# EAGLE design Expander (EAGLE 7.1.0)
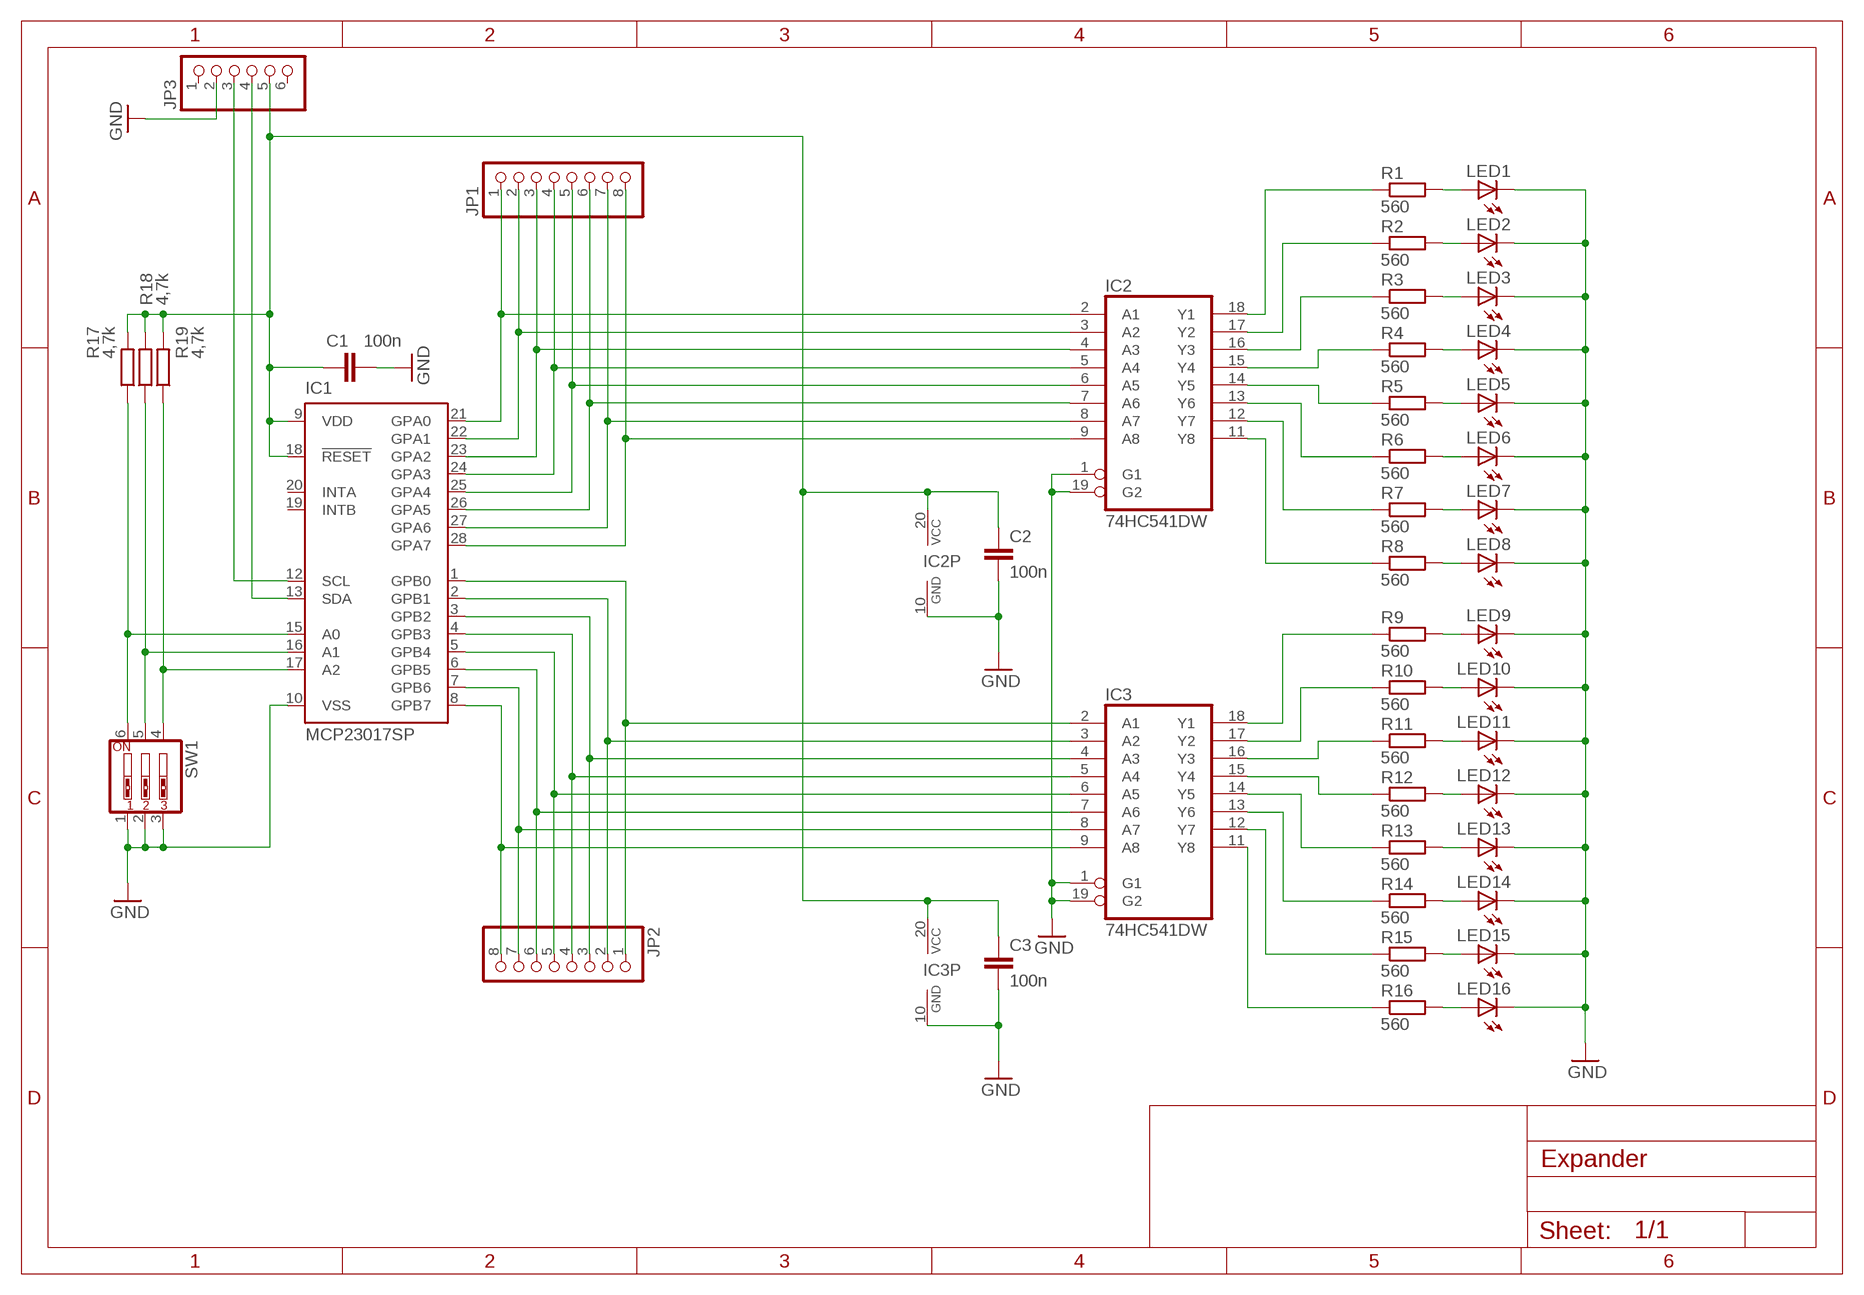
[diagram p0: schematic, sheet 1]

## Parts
C1  100n  C-EUC1206  [C1206]
C2  100n  C-EUC1206  [C1206]
C3  100n  C-EUC1206  [C1206]
IC1  MCP23017SP  [DIL28-3]
IC2  74HC541DW  [SO20W]
IC3  74HC541DW  [SO20W]
JP1  PINHD-1X8  [1X08]
JP2  PINHD-1X8  [1X08]
JP3  PINHD-1X6/90  [1X06/90]
LED1  LEDSMT1206  [1206]
LED2  LEDSMT1206  [1206]
LED3  LEDSMT1206  [1206]
LED4  LEDSMT1206  [1206]
LED5  LEDSMT1206  [1206]
LED6  LEDSMT1206  [1206]
LED7  LEDSMT1206  [1206]
LED8  LEDSMT1206  [1206]
LED9  LEDSMT1206  [1206]
LED10  LEDSMT1206  [1206]
LED11  LEDSMT1206  [1206]
LED12  LEDSMT1206  [1206]
LED13  LEDSMT1206  [1206]
LED14  LEDSMT1206  [1206]
LED15  LEDSMT1206  [1206]
LED16  LEDSMT1206  [1206]
R1  560  R-EU_R1206  [R1206]
R2  560  R-EU_R1206  [R1206]
R3  560  R-EU_R1206  [R1206]
R4  560  R-EU_R1206  [R1206]
R5  560  R-EU_R1206  [R1206]
R6  560  R-EU_R1206  [R1206]
R7  560  R-EU_R1206  [R1206]
R8  560  R-EU_R1206  [R1206]
R9  560  R-EU_R1206  [R1206]
R10  560  R-EU_R1206  [R1206]
R11  560  R-EU_R1206  [R1206]
R12  560  R-EU_R1206  [R1206]
R13  560  R-EU_R1206  [R1206]
R14  560  R-EU_R1206  [R1206]
R15  560  R-EU_R1206  [R1206]
R16  560  R-EU_R1206  [R1206]
R17  4,7k  R-EU_R1206  [R1206]
R18  4,7k  R-EU_R1206  [R1206]
R19  4,7k  R-EU_R1206  [R1206]
SW1  SW_DIP-3  [EDG-03]

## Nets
GND: C1.2 C2.2 C3.2 IC1.10(VSS) IC2.1(G1) IC2.10(GND) IC2.19(G2) IC3.1(G1) IC3.10(GND) IC3.19(G2) JP3.2 LED1.C LED2.C LED3.C LED4.C LED5.C LED6.C LED7.C LED8.C LED9.C LED10.C LED11.C LED12.C LED13.C LED14.C LED15.C LED16.C SW1.1 SW1.2 SW1.3
N$1: IC1.28(GPA7) IC2.9(A8) JP1.8
N$2: IC1.27(GPA6) IC2.8(A7) JP1.7
N$3: IC1.26(GPA5) IC2.7(A6) JP1.6
N$4: IC1.25(GPA4) IC2.6(A5) JP1.5
N$5: IC1.24(GPA3) IC2.5(A4) JP1.4
N$6: IC1.23(GPA2) IC2.4(A3) JP1.3
N$7: IC1.22(GPA1) IC2.3(A2) JP1.2
N$8: IC1.21(GPA0) IC2.2(A1) JP1.1
N$9: IC1.1(GPB0) IC3.2(A1) JP2.1
N$10: IC1.2(GPB1) IC3.3(A2) JP2.2
N$11: IC1.3(GPB2) IC3.4(A3) JP2.3
N$12: IC1.4(GPB3) IC3.5(A4) JP2.4
N$13: IC1.5(GPB4) IC3.6(A5) JP2.5
N$14: IC1.6(GPB5) IC3.7(A6) JP2.6
N$15: IC1.7(GPB6) IC3.8(A7) JP2.7
N$16: IC1.8(GPB7) IC3.9(A8) JP2.8
N$17: LED1.A R1.2
N$18: LED2.A R2.2
N$19: LED3.A R3.2
N$20: LED4.A R4.2
N$21: LED5.A R5.2
N$22: LED6.A R6.2
N$23: LED7.A R7.2
N$24: LED8.A R8.2
N$25: IC2.18(Y1) R1.1
N$26: IC2.17(Y2) R2.1
N$27: IC2.16(Y3) R3.1
N$28: IC2.15(Y4) R4.1
N$29: IC2.14(Y5) R5.1
N$30: IC2.13(Y6) R6.1
N$31: IC2.12(Y7) R7.1
N$32: IC2.11(Y8) R8.1
N$33: IC3.18(Y1) R9.1
N$34: IC3.17(Y2) R10.1
N$35: IC3.16(Y3) R11.1
N$36: IC3.15(Y4) R12.1
N$37: IC3.14(Y5) R13.1
N$38: IC3.13(Y6) R14.1
N$39: IC3.12(Y7) R15.1
N$40: IC3.11(Y8) R16.1
N$41: LED9.A R9.2
N$42: LED10.A R10.2
N$43: LED11.A R11.2
N$44: LED12.A R12.2
N$45: LED13.A R13.2
N$46: LED14.A R14.2
N$47: LED15.A R15.2
N$48: LED16.A R16.2
N$49: IC1.17(A2) R19.1 SW1.4
N$50: IC1.16(A1) R18.1 SW1.5
N$51: IC1.15(A0) R17.1 SW1.6
N$54: IC1.12(SCL) JP3.3
N$55: IC1.13(SDA) JP3.4
N$56: C1.1 C2.1 C3.1 IC1.9(VDD) IC1.18(!RESET) IC2.20(VCC) IC3.20(VCC) JP3.5 R17.2 R18.2 R19.2
Unconnected: IC1.19(INTB) IC1.20(INTA) JP3.1 JP3.6

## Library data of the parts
C1-C3 = rcl:C-EU: CAPACITOR, European symbol
IC1 = microchip:MCP23017: http://ww1.microchip.com/downloads/en/DeviceDoc/21952a.pdf Source: http://ww1.microchip.com/downloads/en/DeviceDoc/21952a.pdf; MF: MICROCHIP; MPN: MCP23017-E/SP; OC_FARNELL: 1332088; OC_NEWARK: 31K2959
IC2 IC3 = 74xx-eu:74*541: Octal BUFFER and LINE DRIVER, 3-state
JP1 JP2 = pinhead:PINHD-1X8: PIN HEADER
JP3 = pinhead:PINHD-1X6: PIN HEADER
LED1-LED16 = led:LED: LED
R1-R19 = resistor:R-EU_: RESISTOR, European symbol
SW1 = special:SW_DIP-3: DIP SWITCH

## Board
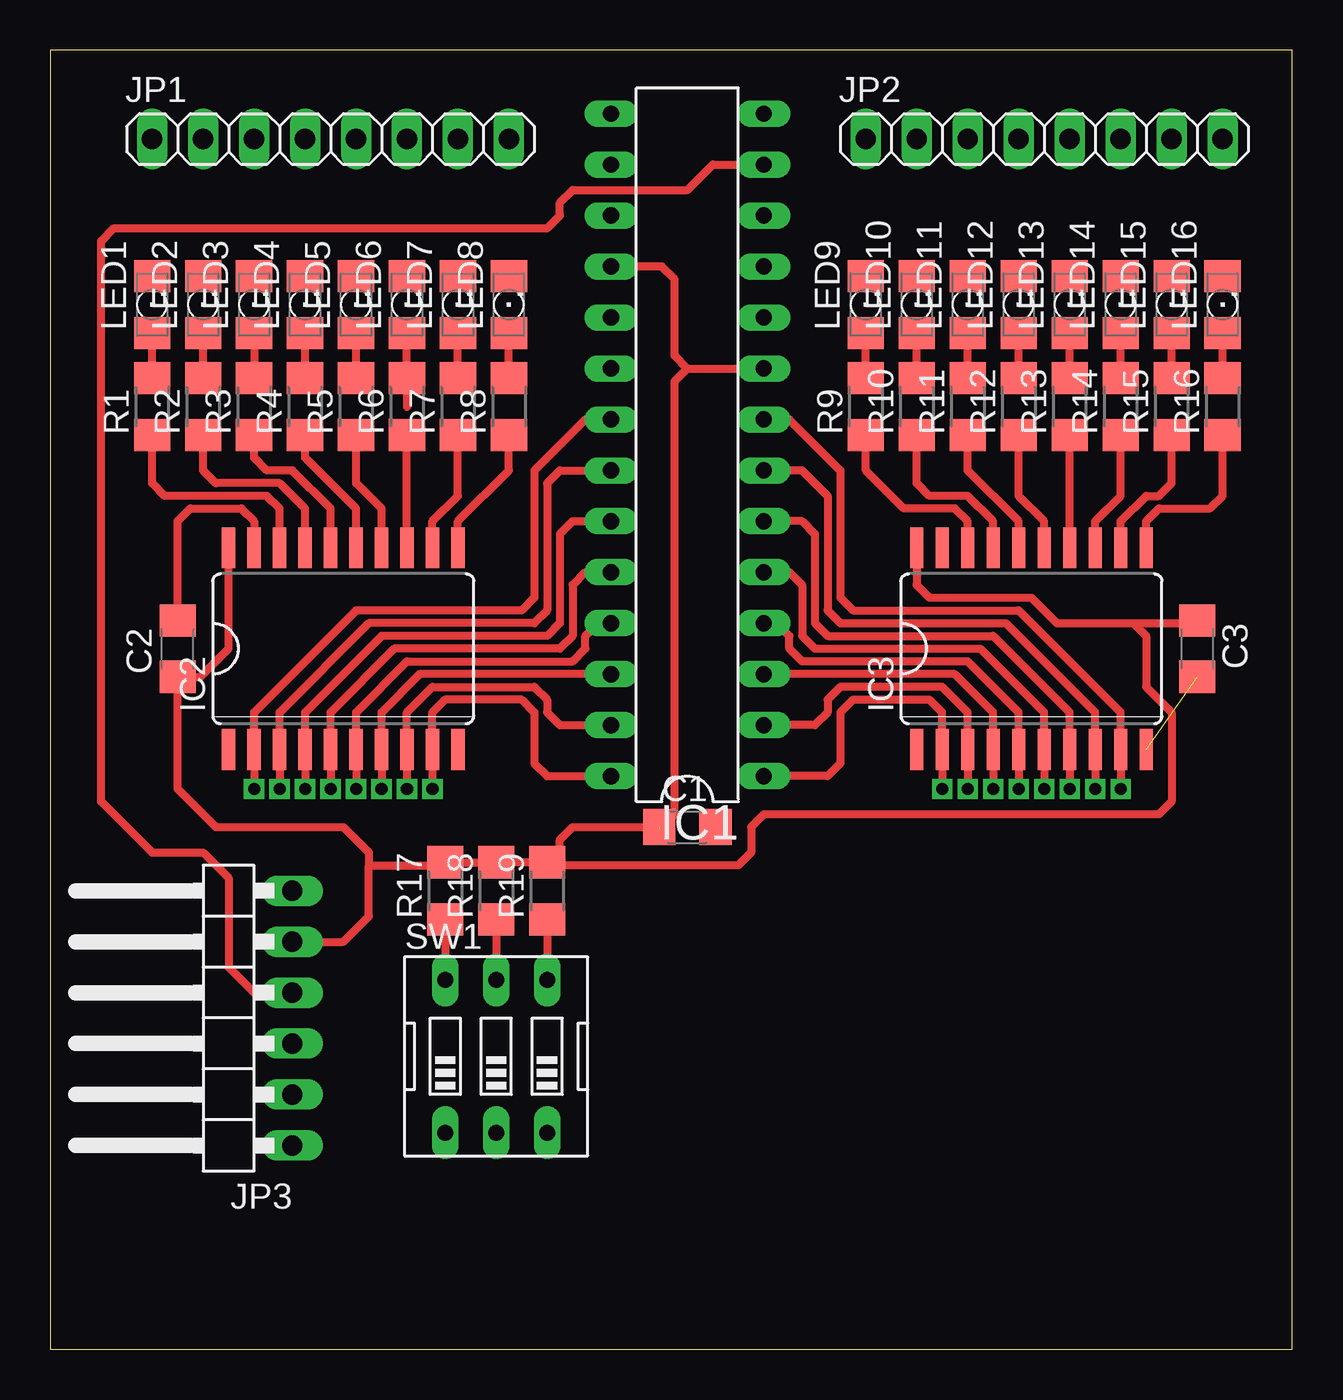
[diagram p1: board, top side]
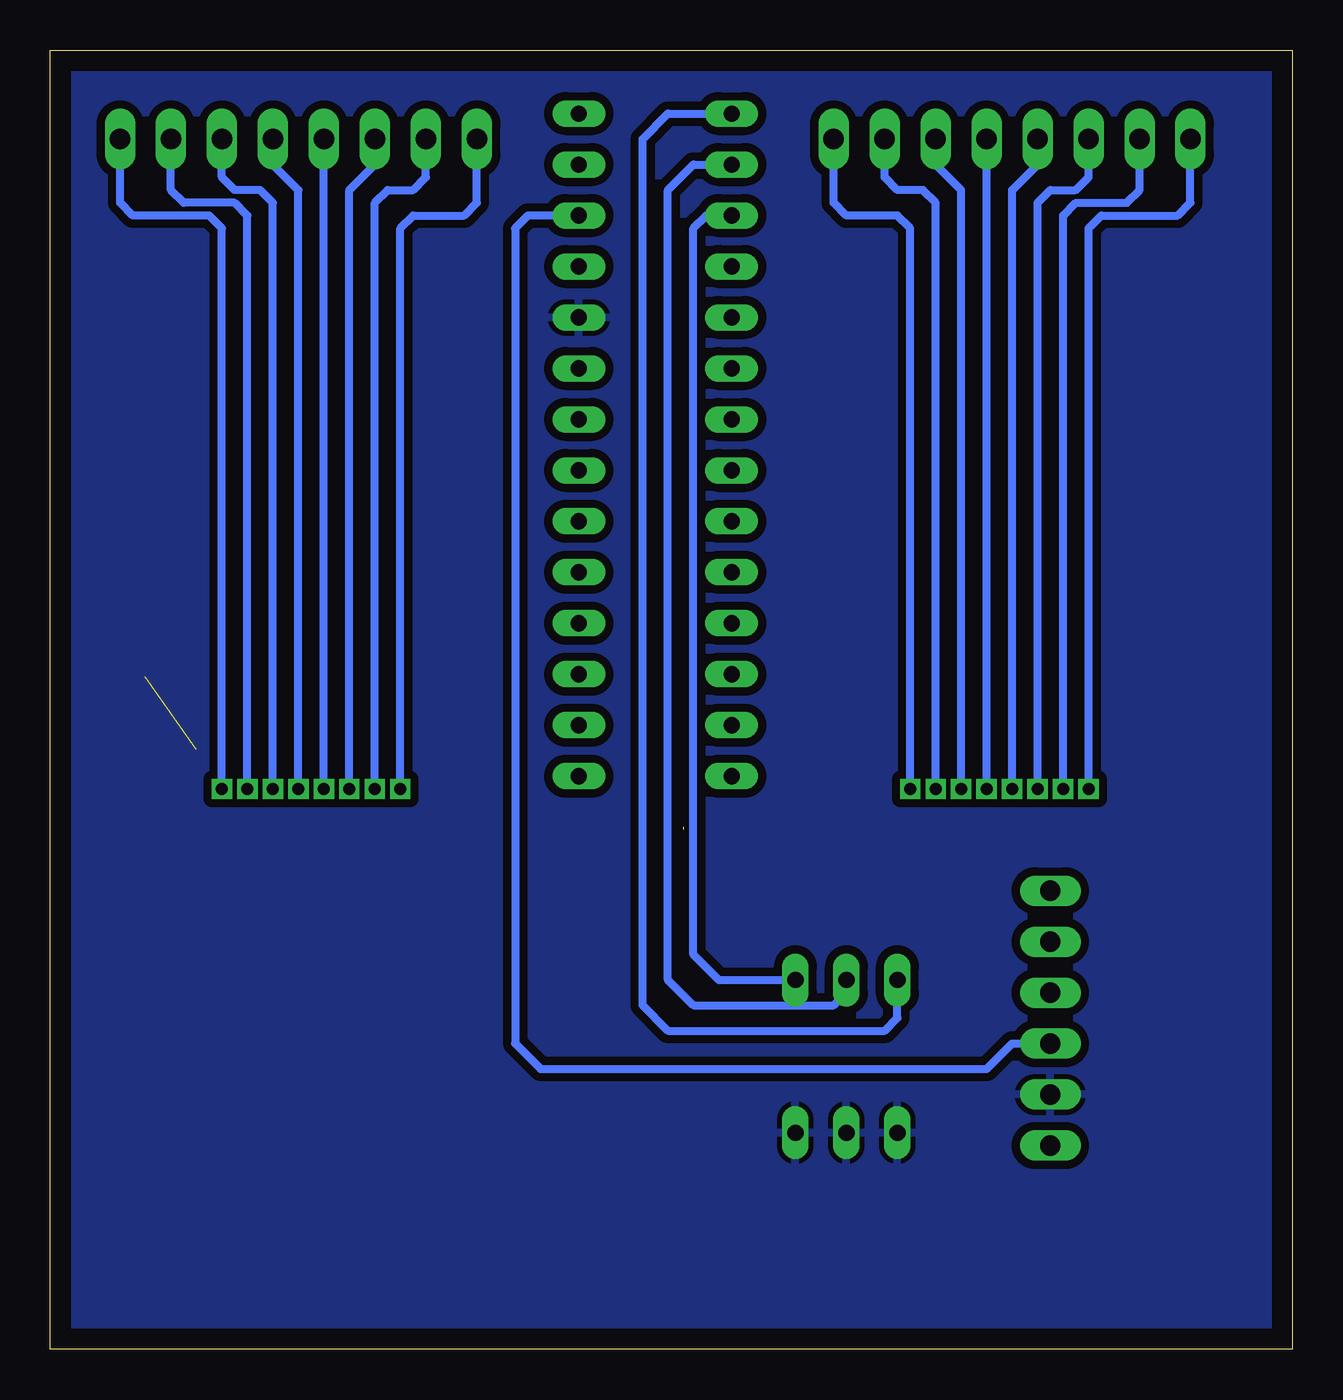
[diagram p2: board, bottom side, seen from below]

Size 61.9 x 64.76 mm. Coordinates in mm from the lower left corner, seen from the top.
Outline: 0,0 61.9,0 61.9,64.76 0,64.76 0,0
Copper layers (1*16): Top 0.035mm / dielectric 1.5mm / Bottom 0.035mm
Design rules "default": minimum track width 10mil, minimum drill 24mil, track to track 8mil, track to pad 8mil, pad to pad 8mil, via to via 8mil, smd to smd 8mil, copper to edge 40mil, drill to drill 8mil, minimum pad ring 10mil, minimum via ring 8mil, stop-mask expansion 4mil, vias tented up to drill 0mil, thermal gap 10mil

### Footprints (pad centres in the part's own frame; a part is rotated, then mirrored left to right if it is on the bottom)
C1206 = smd 1.6 x 1.8: 1 -1.4,0; 2 1.4,0
DIL28-3 = drill 0.813 long: 1 -16.51,-3.81; 2 -13.97,-3.81; 3 -11.43,-3.81; 4 -8.89,-3.81; 5 -6.35,-3.81; 6 -3.81,-3.81; 7 -1.27,-3.81; 8 1.27,-3.81; 9 3.81,-3.81; 10 6.35,-3.81; 11 8.89,-3.81; 12 11.43,-3.81; 13 13.97,-3.81; 14 16.51,-3.81; 15 16.51,3.81; 16 13.97,3.81; 17 11.43,3.81; 18 8.89,3.81; 19 6.35,3.81; 20 3.81,3.81; 21 1.27,3.81; 22 -1.27,3.81; 23 -3.81,3.81; 24 -6.35,3.81; 25 -8.89,3.81; 26 -11.43,3.81; 27 -13.97,3.81; 28 -16.51,3.81
SO20W = smd 0.66 x 2.032: 1 -5.715,-5.029; 2 -4.445,-5.029; 3 -3.175,-5.029; 4 -1.905,-5.029; 5 -0.635,-5.029; 6 0.635,-5.029; 7 1.905,-5.029; 8 3.175,-5.029; 9 4.445,-5.029; 10 5.715,-5.029; 11 5.715,5.029; 12 4.445,5.029; 13 3.175,5.029; 14 1.905,5.029; 15 0.635,5.029; 16 -0.635,5.029; 17 -1.905,5.029; 18 -3.175,5.029; 19 -4.445,5.029; 20 -5.715,5.029
1X08 = drill 1.016 long: 1 -8.89,0; 2 -6.35,0; 3 -3.81,0; 4 -1.27,0; 5 1.27,0; 6 3.81,0; 7 6.35,0; 8 8.89,0
1X06/90 = drill 1.016 long: 1 -6.35,-3.81; 2 -3.81,-3.81; 3 -1.27,-3.81; 4 1.27,-3.81; 5 3.81,-3.81; 6 6.35,-3.81
1206 = smd 1.6 x 1.803: A -1.422,0; C 1.422,0
R1206 = smd 1.6 x 1.803: 1 -1.422,0; 2 1.422,0
EDG-03 = drill 0.813 long: 1 -2.54,-3.81; 2 0,-3.81; 3 2.54,-3.81; 4 2.54,3.81; 5 0,3.81; 6 -2.54,3.81

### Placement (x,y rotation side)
C1  31.75,26.04 0 top
C2  6.35,34.92 90 top
C3  57.15,34.92 270 top
IC1  31.75,45.09 90 top
IC2  14.61,34.92 0 top
IC3  48.9,34.92 0 top
JP1  13.97,60.33 0 top
JP2  49.53,60.33 0 top
JP3  8.26,16.51 90 top
LED1  5.08,52.07 90 top
LED2  7.62,52.07 90 top
LED3  10.16,52.07 90 top
LED4  12.7,52.07 90 top
LED5  15.24,52.07 90 top
LED6  17.78,52.07 90 top
LED7  20.32,52.07 90 top
LED8  22.86,52.07 90 top
LED9  40.64,52.07 90 top
LED10  43.18,52.07 90 top
LED11  45.72,52.07 90 top
LED12  48.26,52.07 90 top
LED13  50.8,52.07 90 top
LED14  53.34,52.07 90 top
LED15  55.88,52.07 90 top
LED16  58.42,52.07 90 top
R1  5.08,46.99 90 top
R2  7.62,46.99 90 top
R3  10.16,46.99 90 top
R4  12.7,46.99 90 top
R5  15.24,46.99 90 top
R6  17.78,46.99 90 top
R7  20.32,46.99 90 top
R8  22.86,46.99 90 top
R9  40.64,46.99 90 top
R10  43.18,46.99 90 top
R11  45.72,46.99 90 top
R12  48.26,46.99 90 top
R13  50.8,46.99 90 top
R14  53.34,46.99 90 top
R15  55.88,46.99 90 top
R16  58.42,46.99 90 top
R17  19.68,22.86 90 top
R18  22.23,22.86 90 top
R19  24.77,22.86 90 top
SW1  22.23,14.61 0 top

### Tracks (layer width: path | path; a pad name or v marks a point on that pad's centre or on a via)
GND  (1 unrouted)
  Top 0.406: C2.2 6.35,41.27 6.99,41.91 9.53,41.91 10.16,41.27 IC2.19
  pour Bottom (isolate 0.406): 0.64,64.14 60.96,64.14 60.96,0.64 0.64,0.64
N$1  (via drill 0.6)
  Top 0.406: IC1.28 24.77,28.57 24.13,29.21 24.13,31.75 23.5,32.38 19.68,32.38 19.05,31.75 IC2.9 v19.05,27.94
  Bottom 0.406: v19.05,27.94 19.05,55.88 19.68,56.52 22.23,56.52 22.86,57.15 JP1.8
N$2  (via drill 0.6)
  Top 0.406: IC1.27 25.4,31.11 24.77,31.75 24.77,32.38 24.13,33.02 19.05,33.02 17.78,31.75 IC2.8 v17.78,27.94
  Bottom 0.406: v17.78,27.94 17.78,57.15 18.41,57.78 19.68,57.78 20.32,58.42 JP1.7
N$3  (via drill 0.6)
  Top 0.406: IC1.26 18.41,33.66 16.51,31.75 IC2.7 v16.51,27.94
  Bottom 0.406: v16.51,27.94 16.51,57.78 17.78,59.05 JP1.6
N$4  (via drill 0.6)
  Top 0.406: IC1.25 27.3,36.2 26.67,35.56 26.67,34.92 26.04,34.29 17.78,34.29 15.24,31.75 IC2.6 v15.24,27.94
  Bottom 0.406: v15.24,27.94 JP1.5
N$5  (via drill 0.6)
  Top 0.406: IC1.24 26.67,38.73 26.04,38.1 26.04,35.56 25.4,34.92 17.14,34.92 13.97,31.75 IC2.5 v13.97,27.94
  Bottom 0.406: v13.97,27.94 13.97,57.78 12.7,59.05 JP1.4
N$6  (via drill 0.6)
  Top 0.406: IC1.23 26.04,41.27 25.4,40.64 25.4,36.2 24.77,35.56 16.51,35.56 12.7,31.75 IC2.4 v12.7,27.94
  Bottom 0.406: v12.7,27.94 12.7,57.15 12.06,57.78 10.79,57.78 10.16,58.42 JP1.3
N$7  (via drill 0.6)
  Top 0.406: IC1.22 25.4,43.81 24.77,43.18 24.77,36.83 24.13,36.2 15.88,36.2 11.43,31.75 IC2.3 v11.43,27.94
  Bottom 0.406: v11.43,27.94 11.43,56.52 10.79,57.15 8.26,57.15 7.62,57.78 JP1.2
N$8  (via drill 0.6)
  Top 0.406: IC1.21 26.67,46.35 24.13,43.81 24.13,37.47 23.5,36.83 15.24,36.83 10.16,31.75 IC2.2 v10.16,27.94
  Bottom 0.406: v10.16,27.94 10.16,55.88 9.53,56.52 5.71,56.52 5.08,57.15 JP1.1
N$9  (via drill 0.6)
  Top 0.406: IC1.1 38.73,28.57 39.37,29.21 39.37,31.75 40.01,32.38 43.81,32.38 44.45,31.75 IC3.2 v44.45,27.94
  Bottom 0.406: v44.45,27.94 44.45,55.88 43.81,56.52 41.27,56.52 40.64,57.15 JP2.1
N$10  (via drill 0.6)
  Top 0.406: IC1.2 38.1,31.11 38.73,31.75 38.73,32.38 39.37,33.02 44.45,33.02 45.72,31.75 IC3.3 v45.72,27.94
  Bottom 0.406: v45.72,27.94 45.72,57.15 45.09,57.78 43.81,57.78 43.18,58.42 JP2.2
N$11  (via drill 0.6)
  Top 0.406: IC1.3 45.09,33.66 46.99,31.75 IC3.4 v46.99,27.94
  Bottom 0.406: v46.99,27.94 46.99,57.78 45.72,59.05 JP2.3
N$12  (via drill 0.6)
  Top 0.406: IC1.4 36.2,36.2 36.83,35.56 36.83,34.92 37.47,34.29 45.72,34.29 48.26,31.75 IC3.5 v48.26,27.94
  Bottom 0.406: v48.26,27.94 JP2.4
N$13  (via drill 0.6)
  Top 0.406: IC1.5 36.83,38.73 37.47,38.1 37.47,35.56 38.1,34.92 46.35,34.92 49.53,31.75 IC3.6 v49.53,27.94
  Bottom 0.406: v49.53,27.94 49.53,57.78 50.8,59.05 JP2.5
N$14  (via drill 0.6)
  Top 0.406: IC1.6 37.47,41.27 38.1,40.64 38.1,36.2 38.73,35.56 46.99,35.56 50.8,31.75 IC3.7 v50.8,27.94
  Bottom 0.406: v50.8,27.94 50.8,57.15 51.44,57.78 52.7,57.78 53.34,58.42 JP2.6
N$15  (via drill 0.6)
  Top 0.406: IC1.7 37.47,43.81 38.73,42.55 38.73,36.83 39.37,36.2 47.62,36.2 52.07,31.75 IC3.8 v52.07,27.94
  Bottom 0.406: v52.07,27.94 52.07,56.52 52.7,57.15 55.24,57.15 55.88,57.78 JP2.7
N$16  (via drill 0.6)
  Top 0.406: IC1.8 36.83,46.35 39.37,43.81 39.37,37.47 40.01,36.83 48.26,36.83 53.34,31.75 IC3.9 v53.34,27.94
  Bottom 0.406: v53.34,27.94 53.34,55.88 53.98,56.52 57.78,56.52 58.42,57.15 JP2.8
N$17
  Top 0.406: R1.2 LED1.A
N$18
  Top 0.406: R2.2 LED2.A
N$19
  Top 0.406: LED3.A R3.2
N$20
  Top 0.406: R4.2 LED4.A
N$21
  Top 0.406: R5.2 LED5.A
N$22
  Top 0.406: 17.78,46.99 R6.2 LED6.A
N$23
  Top 0.406: R7.2 LED7.A
N$24
  Top 0.406: R8.2 LED8.A
N$25
  Top 0.406: IC2.18 11.43,41.91 10.79,42.55 5.71,42.55 5.08,43.18 R1.1
N$26
  Top 0.406: IC2.17 12.7,41.91 11.43,43.18 8.26,43.18 7.62,43.81 R2.1
N$27
  Top 0.406: IC2.16 13.97,41.91 12.06,43.81 10.79,43.81 10.16,44.45 R3.1
N$28
  Top 0.406: IC2.15 15.24,41.91 12.7,44.45 R4.1
N$29
  Top 0.406: IC2.14 16.51,41.91 15.24,43.18 R5.1
N$30
  Top 0.406: IC2.13 R6.1
N$31
  Top 0.406: IC2.12 19.05,41.27 20.32,42.55 R7.1
N$32
  Top 0.406: IC2.11 20.32,41.27 22.86,43.81 R8.1
N$33
  Top 0.406: R9.1 40.64,43.81 42.55,41.91 45.09,41.91 45.72,41.27 IC3.18
N$34
  Top 0.406: IC3.17 46.99,41.27 45.72,42.55 43.81,42.55 43.18,43.18 R10.1
N$35
  Top 0.406: IC3.16 48.26,41.27 45.72,43.81 R11.1
N$36
  Top 0.406: IC3.15 49.53,41.27 48.26,42.55 R12.1
N$37
  Top 0.406: IC3.14 R13.1
N$38
  Top 0.406: IC3.13 52.07,41.27 53.34,42.55 R14.1
N$39
  Top 0.406: IC3.12 53.34,41.27 54.61,42.55 55.24,42.55 55.88,43.18 R15.1
N$40
  Top 0.406: IC3.11 54.61,41.27 55.24,41.91 57.78,41.91 58.42,42.55 R16.1
N$41
  Top 0.406: R9.2 LED9.A
N$42
  Top 0.406: R10.2 LED10.A
N$43
  Top 0.406: R11.2 LED11.A
N$44
  Top 0.406: R12.2 LED12.A
N$45
  Top 0.406: R13.2 LED13.A
N$46
  Top 0.406: R14.2 LED14.A
N$47
  Top 0.406: R15.2 LED15.A
N$48
  Top 0.406: R16.2 LED16.A
N$49
  Top 0.406: R19.1 SW1.4
  Bottom 0.406: IC1.17 29.21,56.52 29.84,55.88 29.84,19.68 28.57,18.41 SW1.4
N$50
  Top 0.406: R18.1 SW1.5
  Bottom 0.406: IC1.16 29.84,59.05 31.11,57.78 31.11,18.41 29.84,17.14 22.86,17.14 22.23,17.78 SW1.5
N$51
  Top 0.406: R17.1 SW1.6
  Bottom 0.406: IC1.15 31.11,61.59 32.38,60.33 32.38,17.14 31.11,15.88 20.32,15.88 19.68,16.51 SW1.6
N$54
  Bottom 0.406: IC1.12 38.1,56.52 38.73,55.88 38.73,15.24 37.47,13.97 15.24,13.97 13.97,15.24 JP3.3
N$55
  Top 0.406: IC1.13 33.02,59.05 31.75,57.78 26.04,57.78 25.4,57.15 25.4,56.52 24.77,55.88 3.17,55.88 2.54,55.24 2.54,27.3 5.08,24.77 7.62,24.77 8.89,23.5 8.89,19.05 10.16,17.78 JP3.4
N$56  (1 unrouted)
  Top 0.406: 53.98,36.2 57.02,36.2 C3.1 | 30.35,25.91 31.11,26.67 31.11,48.26 31.75,48.9 | 31.75,48.9 IC1.9 | 31.75,48.9 31.11,49.53 31.11,53.34 30.48,53.98 IC1.18 | IC2.20 8.89,34.92 7.49,33.52 C2.1 6.35,27.94 8.26,26.04 14.61,26.04 15.88,24.77 15.88,24.13 | IC3.20 43.18,38.1 43.81,37.47 48.9,37.47 50.16,36.2 53.98,36.2 | 53.98,36.2 54.61,35.56 54.61,33.02 55.88,31.75 55.88,27.3 55.24,26.67 35.56,26.67 34.92,26.04 34.92,24.77 34.29,24.13 25.4,24.13 | 25.4,24.13 24.92,24.13 R19.2 R18.2 R17.2 19.53,24.13 15.88,24.13 | 25.4,24.13 25.4,25.4 26.04,26.04 C1.1 | JP3.5 14.61,20.32 15.88,21.59 15.88,24.13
